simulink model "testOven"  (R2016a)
settings: Solver=FixedStepDiscrete  StartTime=0.0  StopTime=8.2  RelTol=1e-3
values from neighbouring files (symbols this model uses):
  t0 = block.DialogPrm(5).Data    [sfun_oven.m]
undefined symbols (not defined in the file or in its folder): newval, oldval

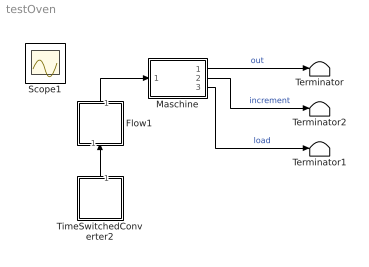
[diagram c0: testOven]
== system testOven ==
  Flow1 : Subsystem
  Maschine : Subsystem
  Terminator : Terminator
  Terminator1 : Terminator
  Terminator2 : Terminator
  TimeSwitchedConverter2 : Subsystem
  Scope1 : Scope
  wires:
  Flow1/1(Out1) -> Maschine/1(in)
  TimeSwitchedConverter2/1(Out1) -> Flow1/1(In1)
  Maschine/1(out) -> Terminator/1  "out"
  Maschine/2(increment) -> Terminator2/1  "increment"
  Maschine/3(load) -> Terminator1/1  "load"

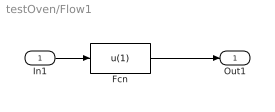
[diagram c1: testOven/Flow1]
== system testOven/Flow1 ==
  In1 : Inport
  Fcn : Fcn  Expr=u(1)
  Out1 : Outport
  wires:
  In1/1 -> Fcn/1
  Fcn/1 -> Out1/1

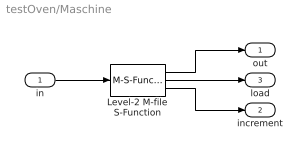
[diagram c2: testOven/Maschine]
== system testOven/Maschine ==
  in : Inport
  Level-2 M-file S-Function : M-S-Function  FunctionName=sfun_oven  Parameters=capacity, cookingtime, initload, dt, t0
  out : Outport
  increment : Outport  Port=2
  load : Outport  Port=3
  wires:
  in/1 -> Level-2 M-file S-Function/1
  Level-2 M-file S-Function/1 -> out/1
  Level-2 M-file S-Function/2 -> load/1
  Level-2 M-file S-Function/3 -> increment/1

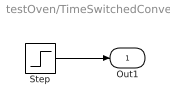
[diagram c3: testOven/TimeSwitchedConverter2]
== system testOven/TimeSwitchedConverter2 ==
  Step : Step  Time=t0  Before=oldval  After=newval
  Out1 : Outport
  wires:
  Step/1 -> Out1/1
